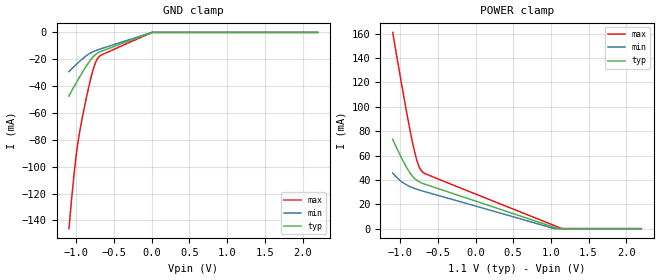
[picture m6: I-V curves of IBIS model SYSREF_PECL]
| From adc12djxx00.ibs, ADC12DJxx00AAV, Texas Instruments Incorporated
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|   Model SYSREF_PECL
[Model]   SYSREF_PECL
Model_type   Input
Vinl = .57
Vinh = 1.33
|   typ   min   max
|   (nom PVT)   (slow PVT)   (fast PVT)
C_comp   0.996p   0.974p   1.029p
[Voltage Range]   1.1   1.05   1.15
[Temperature Range]   27   125   -40
[Power Clamp Reference]   1.1   1.05   1.15
[GND Clamp Reference]   0   0   0
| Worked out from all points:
|   GND clamp passes 1 mA (typ) near -0.04 V on its own axis
[GND Clamp]
|   Voltage   I(typ)   I(min)   I(max)
-1.1V     -47.44mA   -29.21mA   -146.2mA
-1.064V   -43.52mA   -27.17mA   -123.5mA
-1.027V   -39.85mA   -25.18mA   -103mA
-1.001V   -37.26mA   -23.76mA   -90.26mA
-968mV    -34.08mA   -22.03mA   -77.35mA
-888.8mV  -26.76mA   -18.2mA    -53.95mA
-803mV    -19.8mA    -14.99mA   -32.6mA
-753.5mV  -16.8mA    -13.72mA   -23.25mA
-723.8mV  -15.55mA   -13.1mA    -19.72mA
-697.4mV  -14.72mA   -12.58mA   -17.94mA
2.2mV     -24.53uA   -38.05uA   -17.93uA
2.2V      0A         0A         0A
[POWER Clamp]
|   Voltage   I(typ)   I(min)   I(max)
-1.1V     73.18mA    45.59mA    161mA
-997.7mV  59.88mA    39.29mA    124mA
-925.1mV  51.24mA    36.24mA    98.79mA
-872.3mV  45.85mA    34.53mA    81.42mA
-836mV    42.9mA     33.55mA    70.37mA
-796.4mV  40.48mA    32.64mA    59.79mA
-753.5mV  38.65mA    31.79mA    51.36mA
-737mV    38.1mA     31.48mA    49.21mA
-697.4mV  37.03mA    30.77mA    46.16mA
1.045V    1.069mA    11.94uA    2.531mA
1.144V    0A         0A         76.33uA
2.2V      0A         0A         0A
